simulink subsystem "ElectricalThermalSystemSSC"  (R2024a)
settings: Solver=VariableStepAuto  StartTime=0.0  StopTime=10.0  RelTol=1e-3
undefined symbols (not defined in the file): coolant_pipe_D, coolant_valve_D_ratio_max, coolant_valve_D_ratio_min, coolant_valve_displacement, EnvAirTemp, EnvGrvty, PlantThrEstCmpPwr, PlntThrChArea, PlntThrFanMaxSpd, PlntThrFanMechEff, PlntThrFanVolEff, PlntThrHeaterMaxPwr, PlntThrPipeArea, PlntThrPipeDia, PlntThrPmpMaxSpd, PlntThrRadRamEff, PlntThrRefrigAinit, PlntThrTankArea, PlntThrTankVol, PlntThrValDisp, PlntThrValDratioMax, PlntThrValDratioMin, PlntThrValSplMax, ThrmEM1, ThrmEM2, ThrmEM3, ThrmEM4
libraries: fl_lib x148, nesl_utility x61, SimscapeFluids_lib x25, autolibutils x12
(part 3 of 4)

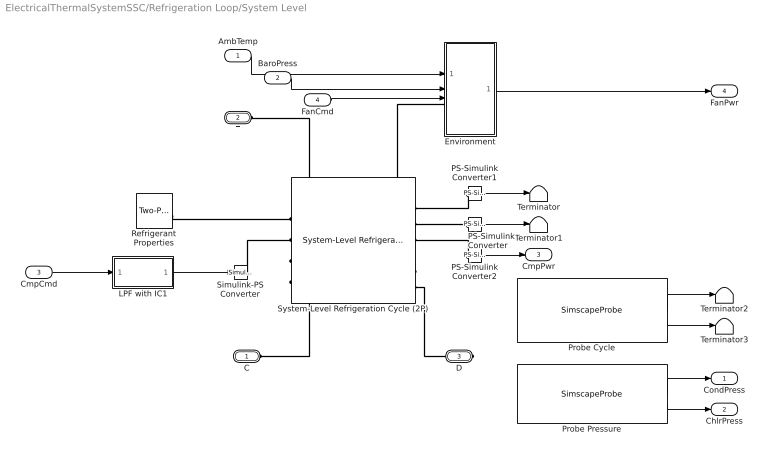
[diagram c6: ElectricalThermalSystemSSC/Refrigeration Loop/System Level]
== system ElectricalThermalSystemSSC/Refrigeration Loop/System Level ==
  AmbTemp : Inport
  BaroPress : Inport  Port=2
  CmpCmd : Inport  Port=3
  FanCmd : Inport  Port=4
  Environment : Subsystem
  LPF with IC1 : Subsystem  mask{wc=0.2, InitCond=0, dataType=off}
      mask prompts: wc "Cutoff frequency, wc [rad/s]"; InitCond "Initial condition, InitCond [same as u]"; dataType "Enforce same input data type"
  PS-Simulink Converter : nesl_utility/PS-Simulink Converter  PhysicalDomain=network_engine_domain  SubClassName=ps_output  LeftPortType=input  RightPortType=output  PseudoPeriodic=off  Frequencies=[]  VectorFormat=inherit  Unit=W  AffineConversion=off
  PS-Simulink Converter1 : nesl_utility/PS-Simulink Converter  PhysicalDomain=network_engine_domain  SubClassName=ps_output  LeftPortType=input  RightPortType=output  PseudoPeriodic=off  Frequencies=[]  VectorFormat=inherit  Unit=W  AffineConversion=off
  PS-Simulink Converter2 : nesl_utility/PS-Simulink Converter  PhysicalDomain=network_engine_domain  SubClassName=ps_output  LeftPortType=input  RightPortType=output  PseudoPeriodic=off  Frequencies=[]  VectorFormat=inherit  Unit=W  AffineConversion=off
  Probe Cycle : SimscapeProbe  BoundBlock=25446  Variables={h_cycle, p_cycle}
  Probe Pressure : SimscapeProbe  BoundBlock=25446  Variables={condenser.refrigerant.p, evaporator.refrigerant.p}
  Refrigerant Properties : SimscapeFluids_lib/Two-Phase Fluid/Utilities/Two-Phase Fluid Predefined Properties (2P)  fluid=fluids.two_phase_fluid.utilities.enum.Fluid.R134a  p_atm=0.101325 MPa  properties_range_check=simscape.enum.assert.action.error  q_rev=0.01 Pa
  Simulink-PS Converter : nesl_utility/Simulink-PS Converter  PhysicalDomain=network_engine_domain  SubClassName=ps_input  LeftPortType=input  RightPortType=output  PseudoPeriodic=off  Frequencies=[]  NoiseDistribution=none  NoiseParameters=[]  Unit=1  AffineConversion=off  FilteringAndDerivatives=provide  SimscapeFilterOrder=1  InputFilterTimeConstant=0.001  UdotUserProvided=0
  System-Level Refrigeration Cycle (2P) : SimscapeFluids_lib/Two-Phase Fluid/Thermodynamic Cycles/System-Level Refrigeration Cycle (2P)  capacity_spec=fluids.two_phase_fluid.thermodynamic_cycles.enum.RefrigerationCycleCapacitySpec.CoolingLoad  Q_cond_nominal=15 kW  Q_evap_nominal=PlntThrCycNomHeatflw kW  mdot_nominal=0.005 kg/s  pressure_spec=fluids.two_phase_fluid.thermodynamic_cycles.enum.RefrigerationCyclePressureSpec.Pressure  p_cond_nominal=PlntThrCycCondRefPin kPa  p_evap_nominal=PlntThrCycChlrRefPin kPa  T_cond_nominal=333.15 K  T_evap_nominal=273.15 K  delta_T_sub_nominal=5 deltaK  delta_T_sup_nominal=10 deltaK  delta_T_sup_static=5 deltaK  performance_spec=fluids.two_phase_fluid.thermodynamic_cycles.enum.RefrigerationCyclePerformanceSpec.COPCooling  COP_nominal=3  comp_eta_s=0.8  comp_eta_v_nominal=0.95  comp_eta_m=0.95  valve_max_fraction=1.5  valve_leak_fraction=1e-6  valve_smoothing_factor=0.01  volume_cond=PlntThrCycCondRefVol m^3  volume_evap=PlntThrCycChlrRefVol m^3  receiver_volume=2 l  receiver_L_init=1 - PlntThrRefrigAinit  nominal_init=true  p_cond_init=refrigerant_p_init MPa  p_evap_init=refrigerant_p_init MPa  h_cond_init=[450, 250] kJ/kg  h_evap_init=[250, 400] kJ/kg  receiver_saturated_init=true  receiver_h_liq_init=500 kJ/kg  receiver_h_vap_init=3500 kJ/kg  cond_domain=fluids.two_phase_fluid.thermodynamic_cycles.enum.RefrigerationCycleFluidDomain.MoistAir  cond_mdot_nominal=PlntThrCycCondAirFlw kg/s  cond_delta_p_nominal=PlntThrCondNomAirDP Pa  cond_pressure_spec=fluids.two_phase_fluid.thermodynamic_cycles.enum.RefrigerationCyclePressureSpec.Pressure  cond_p_in_nominal=PlntThrCondNomPin Pa  cond_T_sat_nominal=400 K  cond_inlet_spec=fluids.two_phase_fluid.thermodynamic_cycles.enum.RefrigerationCycleInletSpec.Enthalpy  cond_T_in_nominal=PlntThrCondNomTin K  cond_h_in_nominal=500 kJ/kg  cond_x_in_nominal=1  cond_inlet_moisture_spec=foundation.enum.moisture_spec.relative_humidity  cond_RH_in_nominal=PlntThrCondNomRelH  cond_x_w_in_nominal=0.01  cond_y_w_in_nominal=0.01  cond_HR_in_nominal=0.01  cond_Tw_in_nominal=287 K  cond_inlet_trace_gas_spec=foundation.enum.trace_gas_spec.mole_fraction  cond_x_g_in_nominal=cabin_CO2_init  cond_y_g_in_nominal=PlntThrCabCO2Init  cond_volume=PlntThrCycCondNomVol m^3  area_Ac=PlntThrCabDucArea m^2  area_Bc=PlntThrCabDucArea m^2  cond_wall_thermal_mass=true  cond_mass_wall=1 kg  cond_cp_wall=890 J/(K*kg)  cond_nominal_init=false  cond_p_init=EnvAbsPrs Pa  cond_energy_spec=foundation.enum.energy_spec.enthalpy  cond_T_init=EnvAirTemp K  cond_x_init=0.5  cond_alpha_init=0.5  cond_h_init=1500 kJ/kg  cond_u_init=1500 kJ/kg  cond_moisture_spec=foundation.enum.moisture_spec.relative_humidity  cond_RH_init=PlntThrCabRelHInit  cond_x_w_init=0.01  cond_y_w_init=0.01  cond_HR_init=0.01  cond_Tw_init=287 K  cond_trace_gas_spec=foundation.enum.trace_gas_spec.mole_fraction  cond_x_g_init=0.001  cond_y_g_init=PlntThrCabCO2Init  cond_T_wall_init=EnvAirTemp K  cond_RH_ws=1  evap_domain=fluids.two_phase_fluid.thermodynamic_cycles.enum.RefrigerationCycleFluidDomain.ThermalLiquid  evap_mdot_nominal=PlntThrCycChlrH2OFlw kg/s  evap_delta_p_nominal=PlntThrCycChlrH2ODP Pa  evap_pressure_spec=fluids.two_phase_fluid.thermodynamic_cycles.enum.RefrigerationCyclePressureSpec.Pressure  evap_p_in_nominal=PlntThrCycChlrH2OPin Pa  evap_T_sat_nominal=400 K  evap_inlet_spec=fluids.two_phase_fluid.thermodynamic_cycles.enum.RefrigerationCycleInletSpec.Enthalpy  evap_T_in_nominal=PlntThrCycChlrH2OTin K  evap_h_in_nominal=500 kJ/kg  evap_x_in_nominal=1  evap_inlet_moisture_spec=foundation.enum.moisture_spec.relative_humidity  evap_RH_in_nominal=0.1  evap_x_w_in_nominal=0.01  evap_y_w_in_nominal=0.01  evap_HR_in_nominal=0.01  evap_Tw_in_nominal=287 K  evap_inlet_trace_gas_spec=foundation.enum.trace_gas_spec.mass_fraction  evap_x_g_in_nominal=0.001  evap_y_g_in_nominal=0.001  evap_volume=PlntThrCycChlrH2OVol m^3  area_Ae=PlntThrPipeArea m^2  area_Be=PlntThrPipeArea m^2  evap_wall_thermal_mass=true  evap_mass_wall=1 kg  evap_cp_wall=890 J/(K*kg)  evap_nominal_init=false  evap_p_init=EnvAbsPrs Pa  evap_energy_spec=foundation.enum.energy_spec.enthalpy  evap_T_init=EnvAirTemp K  evap_x_init=0.5  evap_alpha_init=0.5  evap_h_init=1500 kJ/kg  evap_u_init=1500 kJ/kg  evap_moisture_spec=foundation.enum.moisture_spec.relative_humidity  evap_RH_init=0.5  evap_x_w_init=0.01  evap_y_w_init=0.01  evap_HR_init=0.01  evap_Tw_init=287 K  evap_trace_gas_spec=foundation.enum.trace_gas_spec.mass_fraction  evap_x_g_init=0.001  evap_y_g_init=0.001  evap_T_wall_init=EnvAirTemp K  evap_RH_ws=1  cond_coeff_modify=false  cond_a_liq_refrig=0.023  cond_a_mix_refrig=0.005  cond_a_vap_refrig=0.023  cond_b_refrig=0.8  cond_c_refrig=0.33  cond_a_liq_extfld=0.023  cond_a_mix_extfld=0.005  cond_a_vap_extfld=0.023  cond_a_extfld=0.023  cond_b_extfld=0.8  cond_c_extfld=0.33  evap_coeff_modify=false  evap_a_liq_refrig=0.023  evap_a_mix_refrig=0.005  evap_a_vap_refrig=0.023  evap_b_refrig=0.8  evap_c_refrig=0.33  evap_a_liq_extfld=0.023  evap_a_mix_extfld=0.005  evap_a_vap_extfld=0.023  evap_a_extfld=0.023  evap_b_extfld=0.8  evap_c_extfld=0.33
  Terminator{,1..3} (4 alike) : Terminator
  C : PMIOPort  Side=Left
  T : PMIOPort  Port=2  Side=Left
  D : PMIOPort  Port=3  Side=Right
  CondPress : Outport
  ChlrPress : Outport  Port=2
  CmpPwr : Outport  Port=3
  FanPwr : Outport  Port=4
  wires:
  PS-Simulink Converter2/1 -> CmpPwr/1
  Environment/1(FanPwr) -> FanPwr/1
  FanCmd/1 -> Environment/3(FanCmd)
  AmbTemp/1 -> Environment/1(AmbTemp)
  BaroPress/1 -> Environment/2(BaroPress)
  LPF with IC1/1(y) -> Simulink-PS Converter/1
  Probe Pressure/2 -> ChlrPress/1
  Probe Pressure/1 -> CondPress/1
  Probe Cycle/1 -> Terminator2/1
  Probe Cycle/2 -> Terminator3/1
  CmpCmd/1 -> LPF with IC1/1(u)
  PS-Simulink Converter1/1 -> Terminator/1
  PS-Simulink Converter/1 -> Terminator1/1
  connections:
  PS-Simulink Converter2/LConn1 -- System-Level Refrigeration Cycle (2P)/RConn3
  PS-Simulink Converter1/LConn1 -- System-Level Refrigeration Cycle (2P)/RConn1
  PS-Simulink Converter/LConn1 -- System-Level Refrigeration Cycle (2P)/RConn2
  Simulink-PS Converter/RConn1 -- System-Level Refrigeration Cycle (2P)/LConn2
  C/RConn1 -- System-Level Refrigeration Cycle (2P)/RConn5
  D/RConn1 -- System-Level Refrigeration Cycle (2P)/RConn6
  Environment/LConn1 -- System-Level Refrigeration Cycle (2P)/LConn4
  Refrigerant Properties/RConn1 -- System-Level Refrigeration Cycle (2P)/LConn1
  T/RConn1 -- System-Level Refrigeration Cycle (2P)/LConn3

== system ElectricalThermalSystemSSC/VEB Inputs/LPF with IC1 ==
  u : Inport
  Cont LPF IC : autolibutils/Cont LPF IC  wc=wc  aMode=1  dataType=off
  Initial Condition : Constant  Value=InitCond  SampleTime=-1
  y : Outport
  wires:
  Initial Condition/1 -> Cont LPF IC/2
  u/1 -> Cont LPF IC/1
  Cont LPF IC/1 -> y/1

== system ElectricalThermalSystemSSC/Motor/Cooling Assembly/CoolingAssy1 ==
  CoolEM1 : fl_lib/Thermal/Thermal Elements/Thermal Mass  mass_type=foundation.enum.constant_variable.constant  mass=1 kg  sp_heat=PlntEMCp J/kg/K  mass_min=1e-6 kg  num_ports=foundation.enum.numPorts2.two  m_specify=off  m_priority=High  m=1 kg  m_nominal_specify=off  m_nominal_value=1  m_nominal_unit=kg  T_specify=on  T_priority=High  T=EnvAirTemp K  T_nominal_specify=off  T_nominal_value=1  T_nominal_unit=K  Q_specify=off  Q_priority=None  Q=0 W  Q_nominal_specify=off  Q_nominal_value=1  Q_nominal_unit=W
  Coolant Jacket : SimscapeFluids_lib/Thermal Liquid/Pipes & Fittings/Pipe (TL)  dynamic_compressibility=simscape.enum.onoff.on  inertia=simscape.enum.onoff.off  num_segments=1  pipe_length=PlntThrEMJacLen m  cross_section_geometry=fluids.thermal_liquid.pipes_fittings.enum.CrossSectionGeometry.Custom  pipe_diameter=0.1 m  pipe_inner_diameter=0.05 m  pipe_outer_diameter=0.1 m  pipe_width=0.1 m  pipe_height=0.1 m  pipe_major_axis=0.1 m  pipe_minor_axis=0.05 m  pipe_side=0.1 m  pipe_angle=30 deg  area=PlntThrChArea m^2  Dh=PlntThrChDia m  elevation_spec=foundation.enum.constant_variable.constant  elevation_gain=0 m  gravity_spec=foundation.enum.constant_variable.constant  g=EnvGrvty m/s^2  pressure_loss_spec=fluids.thermal_liquid.pipes_fittings.enum.PressureLossSpec.Haaland  local_pressure_loss_spec=fluids.thermal_liquid.pipes_fittings.enum.LocalLossSpec.AggregateLength  length_add=PlntThrEqLength m  loss_coefficient=0.1  roughness_spec=fluids.thermal_liquid.pipes_fittings.enum.RoughnessSpec.Custom  roughness=1.5e-5 m  Re_friction_TLU=[ 400 1000 1.5e+3 3e+3 4e+3 6e+3 1e+4 2e+4 4e+4 6e+4 1e+5 1e+8 ]  friction_factor_TLU=[ 0.264 0.112 0.07099999999999999 0.0417 0.0387 0.0268 0.025 0.0232 0.0226 0.022 0.0214 0.0214 ]  Re_lam=100  Re_tur=500  shape_factor=64  mdot_nominal=[ 0.1 1 ] kg/s  p_diff_nominal=[ 0.001 0.01 ] MPa  mdot_threshold=1e-6 kg/s  wall_spec=fluids.thermal_liquid.pipes_fittings.enum.wall_spec.rigid  vol_expansion_spec=fluids.thermal_liquid.pipes_fittings.enum.VolumeExpansionSpec.Diameter  area_pressure_gain=1e-6 m^2/MPa  static_pressure_TLU=[.1, 1] MPa  area_pressure_gain_TLU=[1e-05, 1.1e-05] m^2  material_behavior_spec=fluids.thermal_liquid.pipes_fittings.enum.PipeMaterialBehavior.Linear  diameter_pressure_gain=1.2e-6 m/MPa  wall_thickness=0.05 m  elastic_modulus=69 GPa  stress_TLU=[276, 310] MPa  strain_TLU=[.004, .02]  stress_assert_action=simscape.enum.assert.action.none  stress_max=400 MPa  poisson_ratio=0.33  wall_time_constant=0.01 s  thermal_expansion=false  alpha_L_wall=24 um/(deltaK*m)  thermal_expansion_Tref=293.15 K  heat_transfer_spec=fluids.thermal_liquid.pipes_fittings.enum.HeatTransferSpec.DittusBoelter  mdot_nominal_heat=[ 0.1 1 ] kg/s  T_in_nominal=[ 293.15 293.15 ] K  T_out_nominal=[ 300 300 ] K  p_in_nominal_heat=[ 0.101325 0.101325 ] MPa  T_wall_nominal=[ 303.15 303.15 ] K  a_coeff=0.3  b_Re_power=0.8  c_Pr_power=0.33  Nu_lam=3.66  Re_Colburn_TLU=[ 100 150 1000 ]  Colburn_factor_TLU=[ 0.019 0.013 0.002 ]  Re_Nu_TLU=[ 100 150 1000 ]  Pr_Nu_TLU=[ 1 10 ]  Nu_TLU=[ 3.72 4.21; 3.75 4.44; 4.21 7.15 ]  p0_vec=EnvAbsPrs Pa  T0_vec=EnvAirTemp K  mdot0=0.1 kg/s
  PS-Simulink Converter : nesl_utility/PS-Simulink Converter  PhysicalDomain=network_engine_domain  SubClassName=ps_output  LeftPortType=input  RightPortType=output  PseudoPeriodic=off  Frequencies=[]  VectorFormat=1-D array  Unit=K  AffineConversion=on
  Temperature Sensor : fl_lib/Thermal/Thermal Sensors/Temperature Sensor  temperature_measure=foundation.enum.MeasurementReference.difference
  Thermal Reference1 : fl_lib/Thermal/Thermal Elements/Thermal Reference
  H1 : PMIOPort  Side=Right
  A : PMIOPort  Port=2  Side=Left
  B : PMIOPort  Port=3  Side=Right
  EMTemp : Outport
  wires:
  PS-Simulink Converter/1 -> EMTemp/1
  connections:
  Thermal Reference1/LConn1 -- Temperature Sensor/RConn1
  Temperature Sensor/RConn2 -- PS-Simulink Converter/LConn1
  Coolant Jacket/RConn1 -- B/RConn1
  A/RConn1 -- Coolant Jacket/LConn1
  CoolEM1/RConn1 -- Temperature Sensor/LConn1 -- Coolant Jacket/LConn2
  CoolEM1/LConn1 -- H1/RConn1

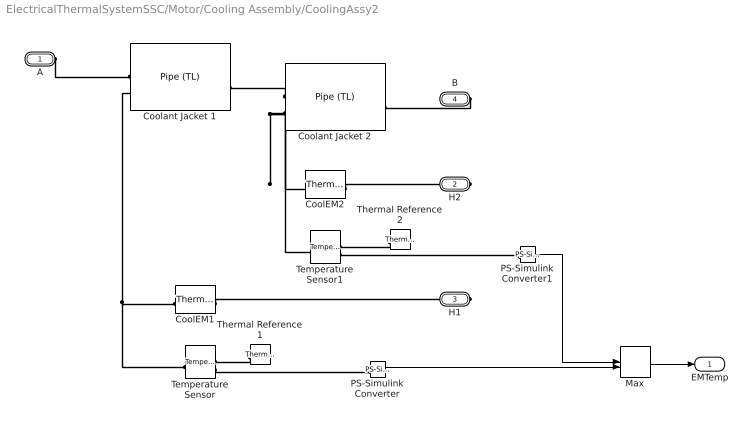
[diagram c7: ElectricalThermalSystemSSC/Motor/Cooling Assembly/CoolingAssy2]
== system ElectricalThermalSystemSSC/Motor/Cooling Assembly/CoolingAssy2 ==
  CoolEM1 : fl_lib/Thermal/Thermal Elements/Thermal Mass  mass_type=foundation.enum.constant_variable.constant  mass=1 kg  sp_heat=PlntEMCp J/kg/K  mass_min=1e-6 kg  num_ports=foundation.enum.numPorts2.two  m_specify=off  m_priority=High  m=1 kg  m_nominal_specify=off  m_nominal_value=1  m_nominal_unit=kg  T_specify=on  T_priority=High  T=EnvAirTemp K  T_nominal_specify=off  T_nominal_value=1  T_nominal_unit=K  Q_specify=off  Q_priority=None  Q=0 W  Q_nominal_specify=off  Q_nominal_value=1  Q_nominal_unit=W
  CoolEM2 : fl_lib/Thermal/Thermal Elements/Thermal Mass  mass_type=foundation.enum.constant_variable.constant  mass=1 kg  sp_heat=PlntEMCp J/kg/K  mass_min=1e-6 kg  num_ports=foundation.enum.numPorts2.two  m_specify=off  m_priority=High  m=1 kg  m_nominal_specify=off  m_nominal_value=1  m_nominal_unit=kg  T_specify=on  T_priority=High  T=EnvAirTemp K  T_nominal_specify=off  T_nominal_value=1  T_nominal_unit=K  Q_specify=off  Q_priority=None  Q=0 W  Q_nominal_specify=off  Q_nominal_value=1  Q_nominal_unit=W
  Coolant Jacket 1 : SimscapeFluids_lib/Thermal Liquid/Pipes & Fittings/Pipe (TL)  dynamic_compressibility=simscape.enum.onoff.on  inertia=simscape.enum.onoff.off  num_segments=1  pipe_length=PlntThrEMJacLen m  cross_section_geometry=fluids.thermal_liquid.pipes_fittings.enum.CrossSectionGeometry.Custom  pipe_diameter=0.1 m  pipe_inner_diameter=0.05 m  pipe_outer_diameter=0.1 m  pipe_width=0.1 m  pipe_height=0.1 m  pipe_major_axis=0.1 m  pipe_minor_axis=0.05 m  pipe_side=0.1 m  pipe_angle=30 deg  area=PlntThrChArea m^2  Dh=PlntThrChDia m  elevation_spec=foundation.enum.constant_variable.constant  elevation_gain=0 m  gravity_spec=foundation.enum.constant_variable.constant  g=EnvGrvty m/s^2  pressure_loss_spec=fluids.thermal_liquid.pipes_fittings.enum.PressureLossSpec.Haaland  local_pressure_loss_spec=fluids.thermal_liquid.pipes_fittings.enum.LocalLossSpec.AggregateLength  length_add=PlntThrEqLength m  loss_coefficient=0.1  roughness_spec=fluids.thermal_liquid.pipes_fittings.enum.RoughnessSpec.Custom  roughness=1.5e-5 m  Re_friction_TLU=[ 400 1000 1.5e+3 3e+3 4e+3 6e+3 1e+4 2e+4 4e+4 6e+4 1e+5 1e+8 ]  friction_factor_TLU=[ 0.264 0.112 0.07099999999999999 0.0417 0.0387 0.0268 0.025 0.0232 0.0226 0.022 0.0214 0.0214 ]  Re_lam=100  Re_tur=500  shape_factor=64  mdot_nominal=[ 0.1 1 ] kg/s  p_diff_nominal=[ 0.001 0.01 ] MPa  mdot_threshold=1e-6 kg/s  wall_spec=fluids.thermal_liquid.pipes_fittings.enum.wall_spec.rigid  vol_expansion_spec=fluids.thermal_liquid.pipes_fittings.enum.VolumeExpansionSpec.Diameter  area_pressure_gain=1e-6 m^2/MPa  static_pressure_TLU=[.1, 1] MPa  area_pressure_gain_TLU=[1e-05, 1.1e-05] m^2  material_behavior_spec=fluids.thermal_liquid.pipes_fittings.enum.PipeMaterialBehavior.Linear  diameter_pressure_gain=1.2e-6 m/MPa  wall_thickness=0.05 m  elastic_modulus=69 GPa  stress_TLU=[276, 310] MPa  strain_TLU=[.004, .02]  stress_assert_action=simscape.enum.assert.action.none  stress_max=400 MPa  poisson_ratio=0.33  wall_time_constant=0.01 s  thermal_expansion=false  alpha_L_wall=24 um/(deltaK*m)  thermal_expansion_Tref=293.15 K  heat_transfer_spec=fluids.thermal_liquid.pipes_fittings.enum.HeatTransferSpec.DittusBoelter  mdot_nominal_heat=[ 0.1 1 ] kg/s  T_in_nominal=[ 293.15 293.15 ] K  T_out_nominal=[ 300 300 ] K  p_in_nominal_heat=[ 0.101325 0.101325 ] MPa  T_wall_nominal=[ 303.15 303.15 ] K  a_coeff=0.3  b_Re_power=0.8  c_Pr_power=0.33  Nu_lam=3.66  Re_Colburn_TLU=[ 100 150 1000 ]  Colburn_factor_TLU=[ 0.019 0.013 0.002 ]  Re_Nu_TLU=[ 100 150 1000 ]  Pr_Nu_TLU=[ 1 10 ]  Nu_TLU=[ 3.72 4.21; 3.75 4.44; 4.21 7.15 ]  p0_vec=EnvAbsPrs Pa  T0_vec=EnvAirTemp K  mdot0=0.1 kg/s
  Coolant Jacket 2 : SimscapeFluids_lib/Thermal Liquid/Pipes & Fittings/Pipe (TL)  dynamic_compressibility=simscape.enum.onoff.on  inertia=simscape.enum.onoff.off  num_segments=1  pipe_length=PlntThrEMJacLen m  cross_section_geometry=fluids.thermal_liquid.pipes_fittings.enum.CrossSectionGeometry.Custom  pipe_diameter=0.1 m  pipe_inner_diameter=0.05 m  pipe_outer_diameter=0.1 m  pipe_width=0.1 m  pipe_height=0.1 m  pipe_major_axis=0.1 m  pipe_minor_axis=0.05 m  pipe_side=0.1 m  pipe_angle=30 deg  area=PlntThrChArea m^2  Dh=PlntThrChDia m  elevation_spec=foundation.enum.constant_variable.constant  elevation_gain=0 m  gravity_spec=foundation.enum.constant_variable.constant  g=EnvGrvty m/s^2  pressure_loss_spec=fluids.thermal_liquid.pipes_fittings.enum.PressureLossSpec.Haaland  local_pressure_loss_spec=fluids.thermal_liquid.pipes_fittings.enum.LocalLossSpec.AggregateLength  length_add=PlntThrEqLength m  loss_coefficient=0.1  roughness_spec=fluids.thermal_liquid.pipes_fittings.enum.RoughnessSpec.Custom  roughness=1.5e-5 m  Re_friction_TLU=[ 400 1000 1.5e+3 3e+3 4e+3 6e+3 1e+4 2e+4 4e+4 6e+4 1e+5 1e+8 ]  friction_factor_TLU=[ 0.264 0.112 0.07099999999999999 0.0417 0.0387 0.0268 0.025 0.0232 0.0226 0.022 0.0214 0.0214 ]  Re_lam=100  Re_tur=500  shape_factor=64  mdot_nominal=[ 0.1 1 ] kg/s  p_diff_nominal=[ 0.001 0.01 ] MPa  mdot_threshold=1e-6 kg/s  wall_spec=fluids.thermal_liquid.pipes_fittings.enum.wall_spec.rigid  vol_expansion_spec=fluids.thermal_liquid.pipes_fittings.enum.VolumeExpansionSpec.Diameter  area_pressure_gain=1e-6 m^2/MPa  static_pressure_TLU=[.1, 1] MPa  area_pressure_gain_TLU=[1e-05, 1.1e-05] m^2  material_behavior_spec=fluids.thermal_liquid.pipes_fittings.enum.PipeMaterialBehavior.Linear  diameter_pressure_gain=1.2e-6 m/MPa  wall_thickness=0.05 m  elastic_modulus=69 GPa  stress_TLU=[276, 310] MPa  strain_TLU=[.004, .02]  stress_assert_action=simscape.enum.assert.action.none  stress_max=400 MPa  poisson_ratio=0.33  wall_time_constant=0.01 s  thermal_expansion=false  alpha_L_wall=24 um/(deltaK*m)  thermal_expansion_Tref=293.15 K  heat_transfer_spec=fluids.thermal_liquid.pipes_fittings.enum.HeatTransferSpec.DittusBoelter  mdot_nominal_heat=[ 0.1 1 ] kg/s  T_in_nominal=[ 293.15 293.15 ] K  T_out_nominal=[ 300 300 ] K  p_in_nominal_heat=[ 0.101325 0.101325 ] MPa  T_wall_nominal=[ 303.15 303.15 ] K  a_coeff=0.3  b_Re_power=0.8  c_Pr_power=0.33  Nu_lam=3.66  Re_Colburn_TLU=[ 100 150 1000 ]  Colburn_factor_TLU=[ 0.019 0.013 0.002 ]  Re_Nu_TLU=[ 100 150 1000 ]  Pr_Nu_TLU=[ 1 10 ]  Nu_TLU=[ 3.72 4.21; 3.75 4.44; 4.21 7.15 ]  p0_vec=EnvAbsPrs Pa  T0_vec=EnvAirTemp K  mdot0=0.1 kg/s
  Max : MinMax  Function=max  Inputs=2
  PS-Simulink Converter : nesl_utility/PS-Simulink Converter  PhysicalDomain=network_engine_domain  SubClassName=ps_output  LeftPortType=input  RightPortType=output  PseudoPeriodic=off  Frequencies=[]  VectorFormat=1-D array  Unit=K  AffineConversion=on
  PS-Simulink Converter1 : nesl_utility/PS-Simulink Converter  PhysicalDomain=network_engine_domain  SubClassName=ps_output  LeftPortType=input  RightPortType=output  PseudoPeriodic=off  Frequencies=[]  VectorFormat=1-D array  Unit=K  AffineConversion=on
  Temperature Sensor : fl_lib/Thermal/Thermal Sensors/Temperature Sensor  temperature_measure=foundation.enum.MeasurementReference.difference
  Temperature Sensor1 : fl_lib/Thermal/Thermal Sensors/Temperature Sensor  temperature_measure=foundation.enum.MeasurementReference.difference
  Thermal Reference1 : fl_lib/Thermal/Thermal Elements/Thermal Reference
  Thermal Reference2 : fl_lib/Thermal/Thermal Elements/Thermal Reference
  A : PMIOPort  Side=Left
  H2 : PMIOPort  Port=2  Side=Right
  H1 : PMIOPort  Port=3  Side=Right
  B : PMIOPort  Port=4  Side=Right
  EMTemp : Outport
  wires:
  PS-Simulink Converter/1 -> Max/2
  PS-Simulink Converter1/1 -> Max/1
  Max/1 -> EMTemp/1
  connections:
  PS-Simulink Converter1/LConn1 -- Temperature Sensor1/RConn2
  Thermal Reference2/LConn1 -- Temperature Sensor1/RConn1
  Coolant Jacket 2/LConn2 -- Temperature Sensor1/LConn1 -- CoolEM2/RConn1
  CoolEM2/LConn1 -- H2/RConn1
  B/RConn1 -- Coolant Jacket 2/RConn1
  Coolant Jacket 2/LConn1 -- Coolant Jacket 1/RConn1
  Thermal Reference1/LConn1 -- Temperature Sensor/RConn1
  Temperature Sensor/RConn2 -- PS-Simulink Converter/LConn1
  A/RConn1 -- Coolant Jacket 1/LConn1
  Temperature Sensor/LConn1 -- Coolant Jacket 1/LConn2 -- CoolEM1/RConn1
  CoolEM1/LConn1 -- H1/RConn1

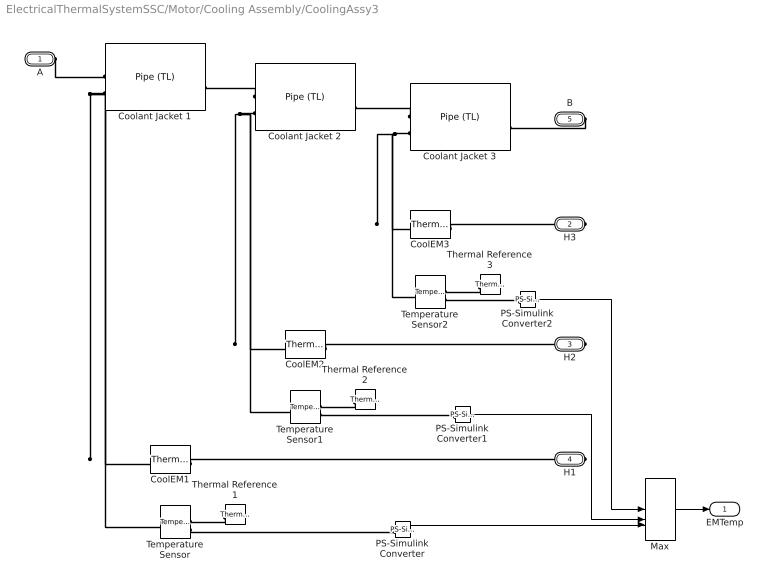
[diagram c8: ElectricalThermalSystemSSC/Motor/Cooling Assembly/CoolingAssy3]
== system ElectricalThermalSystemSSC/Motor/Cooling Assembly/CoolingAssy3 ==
  CoolEM1 : fl_lib/Thermal/Thermal Elements/Thermal Mass  mass_type=foundation.enum.constant_variable.constant  mass=1 kg  sp_heat=PlntEMCp J/kg/K  mass_min=1e-6 kg  num_ports=foundation.enum.numPorts2.two  m_specify=off  m_priority=High  m=1 kg  m_nominal_specify=off  m_nominal_value=1  m_nominal_unit=kg  T_specify=on  T_priority=High  T=EnvAirTemp K  T_nominal_specify=off  T_nominal_value=1  T_nominal_unit=K  Q_specify=off  Q_priority=None  Q=0 W  Q_nominal_specify=off  Q_nominal_value=1  Q_nominal_unit=W
  CoolEM2 : fl_lib/Thermal/Thermal Elements/Thermal Mass  mass_type=foundation.enum.constant_variable.constant  mass=1 kg  sp_heat=PlntEMCp J/kg/K  mass_min=1e-6 kg  num_ports=foundation.enum.numPorts2.two  m_specify=off  m_priority=High  m=1 kg  m_nominal_specify=off  m_nominal_value=1  m_nominal_unit=kg  T_specify=on  T_priority=High  T=EnvAirTemp K  T_nominal_specify=off  T_nominal_value=1  T_nominal_unit=K  Q_specify=off  Q_priority=None  Q=0 W  Q_nominal_specify=off  Q_nominal_value=1  Q_nominal_unit=W
  CoolEM3 : fl_lib/Thermal/Thermal Elements/Thermal Mass  mass_type=foundation.enum.constant_variable.constant  mass=1 kg  sp_heat=PlntEMCp J/kg/K  mass_min=1e-6 kg  num_ports=foundation.enum.numPorts2.two  m_specify=off  m_priority=High  m=1 kg  m_nominal_specify=off  m_nominal_value=1  m_nominal_unit=kg  T_specify=on  T_priority=High  T=EnvAirTemp K  T_nominal_specify=off  T_nominal_value=1  T_nominal_unit=K  Q_specify=off  Q_priority=None  Q=0 W  Q_nominal_specify=off  Q_nominal_value=1  Q_nominal_unit=W
  Coolant Jacket 1 : SimscapeFluids_lib/Thermal Liquid/Pipes & Fittings/Pipe (TL)  dynamic_compressibility=simscape.enum.onoff.on  inertia=simscape.enum.onoff.off  num_segments=1  pipe_length=PlntThrEMJacLen m  cross_section_geometry=fluids.thermal_liquid.pipes_fittings.enum.CrossSectionGeometry.Custom  pipe_diameter=0.1 m  pipe_inner_diameter=0.05 m  pipe_outer_diameter=0.1 m  pipe_width=0.1 m  pipe_height=0.1 m  pipe_major_axis=0.1 m  pipe_minor_axis=0.05 m  pipe_side=0.1 m  pipe_angle=30 deg  area=PlntThrChArea m^2  Dh=PlntThrChDia m  elevation_spec=foundation.enum.constant_variable.constant  elevation_gain=0 m  gravity_spec=foundation.enum.constant_variable.constant  g=EnvGrvty m/s^2  pressure_loss_spec=fluids.thermal_liquid.pipes_fittings.enum.PressureLossSpec.Haaland  local_pressure_loss_spec=fluids.thermal_liquid.pipes_fittings.enum.LocalLossSpec.AggregateLength  length_add=PlntThrEqLength m  loss_coefficient=0.1  roughness_spec=fluids.thermal_liquid.pipes_fittings.enum.RoughnessSpec.Custom  roughness=1.5e-5 m  Re_friction_TLU=[ 400 1000 1.5e+3 3e+3 4e+3 6e+3 1e+4 2e+4 4e+4 6e+4 1e+5 1e+8 ]  friction_factor_TLU=[ 0.264 0.112 0.07099999999999999 0.0417 0.0387 0.0268 0.025 0.0232 0.0226 0.022 0.0214 0.0214 ]  Re_lam=100  Re_tur=500  shape_factor=64  mdot_nominal=[ 0.1 1 ] kg/s  p_diff_nominal=[ 0.001 0.01 ] MPa  mdot_threshold=1e-6 kg/s  wall_spec=fluids.thermal_liquid.pipes_fittings.enum.wall_spec.rigid  vol_expansion_spec=fluids.thermal_liquid.pipes_fittings.enum.VolumeExpansionSpec.Diameter  area_pressure_gain=1e-6 m^2/MPa  static_pressure_TLU=[.1, 1] MPa  area_pressure_gain_TLU=[1e-05, 1.1e-05] m^2  material_behavior_spec=fluids.thermal_liquid.pipes_fittings.enum.PipeMaterialBehavior.Linear  diameter_pressure_gain=1.2e-6 m/MPa  wall_thickness=0.05 m  elastic_modulus=69 GPa  stress_TLU=[276, 310] MPa  strain_TLU=[.004, .02]  stress_assert_action=simscape.enum.assert.action.none  stress_max=400 MPa  poisson_ratio=0.33  wall_time_constant=0.01 s  thermal_expansion=false  alpha_L_wall=24 um/(deltaK*m)  thermal_expansion_Tref=293.15 K  heat_transfer_spec=fluids.thermal_liquid.pipes_fittings.enum.HeatTransferSpec.DittusBoelter  mdot_nominal_heat=[ 0.1 1 ] kg/s  T_in_nominal=[ 293.15 293.15 ] K  T_out_nominal=[ 300 300 ] K  p_in_nominal_heat=[ 0.101325 0.101325 ] MPa  T_wall_nominal=[ 303.15 303.15 ] K  a_coeff=0.3  b_Re_power=0.8  c_Pr_power=0.33  Nu_lam=3.66  Re_Colburn_TLU=[ 100 150 1000 ]  Colburn_factor_TLU=[ 0.019 0.013 0.002 ]  Re_Nu_TLU=[ 100 150 1000 ]  Pr_Nu_TLU=[ 1 10 ]  Nu_TLU=[ 3.72 4.21; 3.75 4.44; 4.21 7.15 ]  p0_vec=EnvAbsPrs Pa  T0_vec=EnvAirTemp K  mdot0=0.1 kg/s
  Coolant Jacket 2 : SimscapeFluids_lib/Thermal Liquid/Pipes & Fittings/Pipe (TL)  dynamic_compressibility=simscape.enum.onoff.on  inertia=simscape.enum.onoff.off  num_segments=1  pipe_length=PlntThrEMJacLen m  cross_section_geometry=fluids.thermal_liquid.pipes_fittings.enum.CrossSectionGeometry.Custom  pipe_diameter=0.1 m  pipe_inner_diameter=0.05 m  pipe_outer_diameter=0.1 m  pipe_width=0.1 m  pipe_height=0.1 m  pipe_major_axis=0.1 m  pipe_minor_axis=0.05 m  pipe_side=0.1 m  pipe_angle=30 deg  area=PlntThrChArea m^2  Dh=PlntThrChDia m  elevation_spec=foundation.enum.constant_variable.constant  elevation_gain=0 m  gravity_spec=foundation.enum.constant_variable.constant  g=EnvGrvty m/s^2  pressure_loss_spec=fluids.thermal_liquid.pipes_fittings.enum.PressureLossSpec.Haaland  local_pressure_loss_spec=fluids.thermal_liquid.pipes_fittings.enum.LocalLossSpec.AggregateLength  length_add=PlntThrEqLength m  loss_coefficient=0.1  roughness_spec=fluids.thermal_liquid.pipes_fittings.enum.RoughnessSpec.Custom  roughness=1.5e-5 m  Re_friction_TLU=[ 400 1000 1.5e+3 3e+3 4e+3 6e+3 1e+4 2e+4 4e+4 6e+4 1e+5 1e+8 ]  friction_factor_TLU=[ 0.264 0.112 0.07099999999999999 0.0417 0.0387 0.0268 0.025 0.0232 0.0226 0.022 0.0214 0.0214 ]  Re_lam=100  Re_tur=500  shape_factor=64  mdot_nominal=[ 0.1 1 ] kg/s  p_diff_nominal=[ 0.001 0.01 ] MPa  mdot_threshold=1e-6 kg/s  wall_spec=fluids.thermal_liquid.pipes_fittings.enum.wall_spec.rigid  vol_expansion_spec=fluids.thermal_liquid.pipes_fittings.enum.VolumeExpansionSpec.Diameter  area_pressure_gain=1e-6 m^2/MPa  static_pressure_TLU=[.1, 1] MPa  area_pressure_gain_TLU=[1e-05, 1.1e-05] m^2  material_behavior_spec=fluids.thermal_liquid.pipes_fittings.enum.PipeMaterialBehavior.Linear  diameter_pressure_gain=1.2e-6 m/MPa  wall_thickness=0.05 m  elastic_modulus=69 GPa  stress_TLU=[276, 310] MPa  strain_TLU=[.004, .02]  stress_assert_action=simscape.enum.assert.action.none  stress_max=400 MPa  poisson_ratio=0.33  wall_time_constant=0.01 s  thermal_expansion=false  alpha_L_wall=24 um/(deltaK*m)  thermal_expansion_Tref=293.15 K  heat_transfer_spec=fluids.thermal_liquid.pipes_fittings.enum.HeatTransferSpec.DittusBoelter  mdot_nominal_heat=[ 0.1 1 ] kg/s  T_in_nominal=[ 293.15 293.15 ] K  T_out_nominal=[ 300 300 ] K  p_in_nominal_heat=[ 0.101325 0.101325 ] MPa  T_wall_nominal=[ 303.15 303.15 ] K  a_coeff=0.3  b_Re_power=0.8  c_Pr_power=0.33  Nu_lam=3.66  Re_Colburn_TLU=[ 100 150 1000 ]  Colburn_factor_TLU=[ 0.019 0.013 0.002 ]  Re_Nu_TLU=[ 100 150 1000 ]  Pr_Nu_TLU=[ 1 10 ]  Nu_TLU=[ 3.72 4.21; 3.75 4.44; 4.21 7.15 ]  p0_vec=EnvAbsPrs Pa  T0_vec=EnvAirTemp K  mdot0=0.1 kg/s
  Coolant Jacket 3 : SimscapeFluids_lib/Thermal Liquid/Pipes & Fittings/Pipe (TL)  dynamic_compressibility=simscape.enum.onoff.on  inertia=simscape.enum.onoff.off  num_segments=1  pipe_length=PlntThrEMJacLen m  cross_section_geometry=fluids.thermal_liquid.pipes_fittings.enum.CrossSectionGeometry.Custom  pipe_diameter=0.1 m  pipe_inner_diameter=0.05 m  pipe_outer_diameter=0.1 m  pipe_width=0.1 m  pipe_height=0.1 m  pipe_major_axis=0.1 m  pipe_minor_axis=0.05 m  pipe_side=0.1 m  pipe_angle=30 deg  area=PlntThrChArea m^2  Dh=PlntThrChDia m  elevation_spec=foundation.enum.constant_variable.constant  elevation_gain=0 m  gravity_spec=foundation.enum.constant_variable.constant  g=EnvGrvty m/s^2  pressure_loss_spec=fluids.thermal_liquid.pipes_fittings.enum.PressureLossSpec.Haaland  local_pressure_loss_spec=fluids.thermal_liquid.pipes_fittings.enum.LocalLossSpec.AggregateLength  length_add=PlntThrEqLength m  loss_coefficient=0.1  roughness_spec=fluids.thermal_liquid.pipes_fittings.enum.RoughnessSpec.Custom  roughness=1.5e-5 m  Re_friction_TLU=[ 400 1000 1.5e+3 3e+3 4e+3 6e+3 1e+4 2e+4 4e+4 6e+4 1e+5 1e+8 ]  friction_factor_TLU=[ 0.264 0.112 0.07099999999999999 0.0417 0.0387 0.0268 0.025 0.0232 0.0226 0.022 0.0214 0.0214 ]  Re_lam=100  Re_tur=500  shape_factor=64  mdot_nominal=[ 0.1 1 ] kg/s  p_diff_nominal=[ 0.001 0.01 ] MPa  mdot_threshold=1e-6 kg/s  wall_spec=fluids.thermal_liquid.pipes_fittings.enum.wall_spec.rigid  vol_expansion_spec=fluids.thermal_liquid.pipes_fittings.enum.VolumeExpansionSpec.Diameter  area_pressure_gain=1e-6 m^2/MPa  static_pressure_TLU=[.1, 1] MPa  area_pressure_gain_TLU=[1e-05, 1.1e-05] m^2  material_behavior_spec=fluids.thermal_liquid.pipes_fittings.enum.PipeMaterialBehavior.Linear  diameter_pressure_gain=1.2e-6 m/MPa  wall_thickness=0.05 m  elastic_modulus=69 GPa  stress_TLU=[276, 310] MPa  strain_TLU=[.004, .02]  stress_assert_action=simscape.enum.assert.action.none  stress_max=400 MPa  poisson_ratio=0.33  wall_time_constant=0.01 s  thermal_expansion=false  alpha_L_wall=24 um/(deltaK*m)  thermal_expansion_Tref=293.15 K  heat_transfer_spec=fluids.thermal_liquid.pipes_fittings.enum.HeatTransferSpec.DittusBoelter  mdot_nominal_heat=[ 0.1 1 ] kg/s  T_in_nominal=[ 293.15 293.15 ] K  T_out_nominal=[ 300 300 ] K  p_in_nominal_heat=[ 0.101325 0.101325 ] MPa  T_wall_nominal=[ 303.15 303.15 ] K  a_coeff=0.3  b_Re_power=0.8  c_Pr_power=0.33  Nu_lam=3.66  Re_Colburn_TLU=[ 100 150 1000 ]  Colburn_factor_TLU=[ 0.019 0.013 0.002 ]  Re_Nu_TLU=[ 100 150 1000 ]  Pr_Nu_TLU=[ 1 10 ]  Nu_TLU=[ 3.72 4.21; 3.75 4.44; 4.21 7.15 ]  p0_vec=EnvAbsPrs Pa  T0_vec=EnvAirTemp K  mdot0=0.1 kg/s
  Max : MinMax  Function=max  Inputs=3
  PS-Simulink Converter : nesl_utility/PS-Simulink Converter  PhysicalDomain=network_engine_domain  SubClassName=ps_output  LeftPortType=input  RightPortType=output  PseudoPeriodic=off  Frequencies=[]  VectorFormat=1-D array  Unit=K  AffineConversion=on
  PS-Simulink Converter1 : nesl_utility/PS-Simulink Converter  PhysicalDomain=network_engine_domain  SubClassName=ps_output  LeftPortType=input  RightPortType=output  PseudoPeriodic=off  Frequencies=[]  VectorFormat=1-D array  Unit=K  AffineConversion=on
  PS-Simulink Converter2 : nesl_utility/PS-Simulink Converter  PhysicalDomain=network_engine_domain  SubClassName=ps_output  LeftPortType=input  RightPortType=output  PseudoPeriodic=off  Frequencies=[]  VectorFormat=1-D array  Unit=K  AffineConversion=on
  Temperature Sensor : fl_lib/Thermal/Thermal Sensors/Temperature Sensor  temperature_measure=foundation.enum.MeasurementReference.difference
  Temperature Sensor1 : fl_lib/Thermal/Thermal Sensors/Temperature Sensor  temperature_measure=foundation.enum.MeasurementReference.difference
  Temperature Sensor2 : fl_lib/Thermal/Thermal Sensors/Temperature Sensor  temperature_measure=foundation.enum.MeasurementReference.difference
  Thermal Reference1 : fl_lib/Thermal/Thermal Elements/Thermal Reference
  Thermal Reference2 : fl_lib/Thermal/Thermal Elements/Thermal Reference
  Thermal Reference3 : fl_lib/Thermal/Thermal Elements/Thermal Reference
  A : PMIOPort  Side=Left
  H3 : PMIOPort  Port=2  Side=Right
  H2 : PMIOPort  Port=3  Side=Right
  H1 : PMIOPort  Port=4  Side=Right
  B : PMIOPort  Port=5  Side=Right
  EMTemp : Outport
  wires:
  PS-Simulink Converter2/1 -> Max/1
  PS-Simulink Converter1/1 -> Max/2
  PS-Simulink Converter/1 -> Max/3
  Max/1 -> EMTemp/1
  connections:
  Coolant Jacket 3/LConn2 -- Temperature Sensor2/LConn1 -- CoolEM3/RConn1
  B/RConn1 -- Coolant Jacket 3/RConn1
  Coolant Jacket 3/LConn1 -- Coolant Jacket 2/RConn1
  Thermal Reference3/LConn1 -- Temperature Sensor2/RConn1
  PS-Simulink Converter2/LConn1 -- Temperature Sensor2/RConn2
  CoolEM3/LConn1 -- H3/RConn1
  PS-Simulink Converter1/LConn1 -- Temperature Sensor1/RConn2
  Thermal Reference2/LConn1 -- Temperature Sensor1/RConn1
  Coolant Jacket 2/LConn2 -- Temperature Sensor1/LConn1 -- CoolEM2/RConn1
  CoolEM2/LConn1 -- H2/RConn1
  Coolant Jacket 2/LConn1 -- Coolant Jacket 1/RConn1
  Thermal Reference1/LConn1 -- Temperature Sensor/RConn1
  Temperature Sensor/RConn2 -- PS-Simulink Converter/LConn1
  A/RConn1 -- Coolant Jacket 1/LConn1
  Coolant Jacket 1/LConn2 -- CoolEM1/RConn1 -- Temperature Sensor/LConn1
  CoolEM1/LConn1 -- H1/RConn1

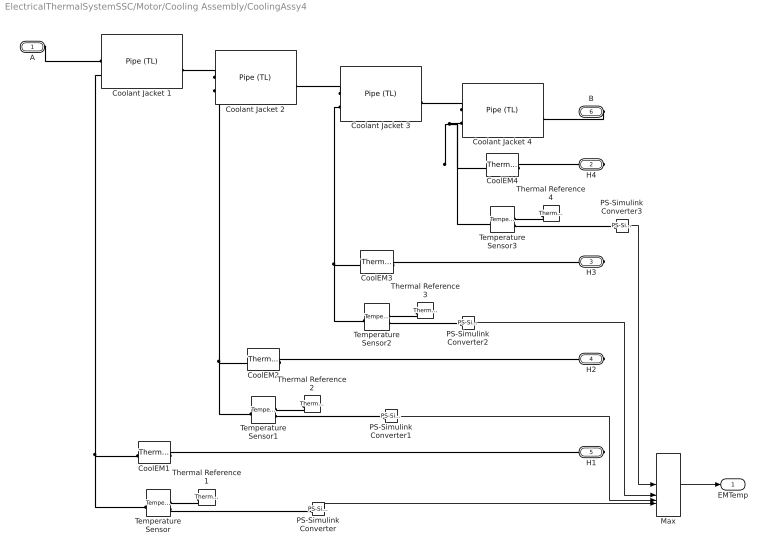
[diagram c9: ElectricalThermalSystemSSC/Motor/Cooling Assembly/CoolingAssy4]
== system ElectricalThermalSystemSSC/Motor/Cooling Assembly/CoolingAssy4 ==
  CoolEM{1..4} (4 alike) : fl_lib/Thermal/Thermal Elements/Thermal Mass  mass_type=foundation.enum.constant_variable.constant  mass=1 kg  sp_heat=PlntEMCp J/kg/K  mass_min=1e-6 kg  num_ports=foundation.enum.numPorts2.two  m_specify=off  m_priority=High  m=1 kg  m_nominal_specify=off  m_nominal_value=1  m_nominal_unit=kg  T_specify=on  T_priority=High  T=EnvAirTemp K  T_nominal_specify=off  T_nominal_value=1  T_nominal_unit=K  Q_specify=off  Q_priority=None  Q=0 W  Q_nominal_specify=off  Q_nominal_value=1  Q_nominal_unit=W
  Coolant Jacket {1..4} (4 alike) : SimscapeFluids_lib/Thermal Liquid/Pipes & Fittings/Pipe (TL)  dynamic_compressibility=simscape.enum.onoff.on  inertia=simscape.enum.onoff.off  num_segments=1  pipe_length=PlntThrEMJacLen m  cross_section_geometry=fluids.thermal_liquid.pipes_fittings.enum.CrossSectionGeometry.Custom  pipe_diameter=0.1 m  pipe_inner_diameter=0.05 m  pipe_outer_diameter=0.1 m  pipe_width=0.1 m  pipe_height=0.1 m  pipe_major_axis=0.1 m  pipe_minor_axis=0.05 m  pipe_side=0.1 m  pipe_angle=30 deg  area=PlntThrChArea m^2  Dh=PlntThrChDia m  elevation_spec=foundation.enum.constant_variable.constant  elevation_gain=0 m  gravity_spec=foundation.enum.constant_variable.constant  g=EnvGrvty m/s^2  pressure_loss_spec=fluids.thermal_liquid.pipes_fittings.enum.PressureLossSpec.Haaland  local_pressure_loss_spec=fluids.thermal_liquid.pipes_fittings.enum.LocalLossSpec.AggregateLength  length_add=PlntThrEqLength m  loss_coefficient=0.1  roughness_spec=fluids.thermal_liquid.pipes_fittings.enum.RoughnessSpec.Custom  roughness=1.5e-5 m  Re_friction_TLU=[ 400 1000 1.5e+3 3e+3 4e+3 6e+3 1e+4 2e+4 4e+4 6e+4 1e+5 1e+8 ]  friction_factor_TLU=[ 0.264 0.112 0.07099999999999999 0.0417 0.0387 0.0268 0.025 0.0232 0.0226 0.022 0.0214 0.0214 ]  Re_lam=100  Re_tur=500  shape_factor=64  mdot_nominal=[ 0.1 1 ] kg/s  p_diff_nominal=[ 0.001 0.01 ] MPa  mdot_threshold=1e-6 kg/s  wall_spec=fluids.thermal_liquid.pipes_fittings.enum.wall_spec.rigid  vol_expansion_spec=fluids.thermal_liquid.pipes_fittings.enum.VolumeExpansionSpec.Diameter  area_pressure_gain=1e-6 m^2/MPa  static_pressure_TLU=[.1, 1] MPa  area_pressure_gain_TLU=[1e-05, 1.1e-05] m^2  material_behavior_spec=fluids.thermal_liquid.pipes_fittings.enum.PipeMaterialBehavior.Linear  diameter_pressure_gain=1.2e-6 m/MPa  wall_thickness=0.05 m  elastic_modulus=69 GPa  stress_TLU=[276, 310] MPa  strain_TLU=[.004, .02]  stress_assert_action=simscape.enum.assert.action.none  stress_max=400 MPa  poisson_ratio=0.33  wall_time_constant=0.01 s  thermal_expansion=false  alpha_L_wall=24 um/(deltaK*m)  thermal_expansion_Tref=293.15 K  heat_transfer_spec=fluids.thermal_liquid.pipes_fittings.enum.HeatTransferSpec.DittusBoelter  mdot_nominal_heat=[ 0.1 1 ] kg/s  T_in_nominal=[ 293.15 293.15 ] K  T_out_nominal=[ 300 300 ] K  p_in_nominal_heat=[ 0.101325 0.101325 ] MPa  T_wall_nominal=[ 303.15 303.15 ] K  a_coeff=0.3  b_Re_power=0.8  c_Pr_power=0.33  Nu_lam=3.66  Re_Colburn_TLU=[ 100 150 1000 ]  Colburn_factor_TLU=[ 0.019 0.013 0.002 ]  Re_Nu_TLU=[ 100 150 1000 ]  Pr_Nu_TLU=[ 1 10 ]  Nu_TLU=[ 3.72 4.21; 3.75 4.44; 4.21 7.15 ]  p0_vec=EnvAbsPrs Pa  T0_vec=EnvAirTemp K  mdot0=0.1 kg/s
  Max : MinMax  Function=max  Inputs=4
  PS-Simulink Converter{,1..3} (4 alike) : nesl_utility/PS-Simulink Converter  PhysicalDomain=network_engine_domain  SubClassName=ps_output  LeftPortType=input  RightPortType=output  PseudoPeriodic=off  Frequencies=[]  VectorFormat=1-D array  Unit=K  AffineConversion=on
  Temperature Sensor{,1..3} (4 alike) : fl_lib/Thermal/Thermal Sensors/Temperature Sensor  temperature_measure=foundation.enum.MeasurementReference.difference
  Thermal Reference{1..4} (4 alike) : fl_lib/Thermal/Thermal Elements/Thermal Reference
  A : PMIOPort  Side=Left
  H4 : PMIOPort  Port=2  Side=Right
  H3 : PMIOPort  Port=3  Side=Right
  H2 : PMIOPort  Port=4  Side=Right
  H1 : PMIOPort  Port=5  Side=Right
  B : PMIOPort  Port=6  Side=Right
  EMTemp : Outport
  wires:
  PS-Simulink Converter3/1 -> Max/1
  PS-Simulink Converter2/1 -> Max/2
  PS-Simulink Converter1/1 -> Max/3
  PS-Simulink Converter/1 -> Max/4
  Max/1 -> EMTemp/1
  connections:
  Coolant Jacket 4/LConn2 -- CoolEM4/RConn1 -- Temperature Sensor3/LConn1
  PS-Simulink Converter3/LConn1 -- Temperature Sensor3/RConn2
  Thermal Reference4/LConn1 -- Temperature Sensor3/RConn1
  CoolEM4/LConn1 -- H4/RConn1
  B/RConn1 -- Coolant Jacket 4/RConn1
  Coolant Jacket 4/LConn1 -- Coolant Jacket 3/RConn1
  Temperature Sensor2/LConn1 -- Coolant Jacket 3/LConn2 -- CoolEM3/RConn1
  Coolant Jacket 3/LConn1 -- Coolant Jacket 2/RConn1
  Thermal Reference3/LConn1 -- Temperature Sensor2/RConn1
  PS-Simulink Converter2/LConn1 -- Temperature Sensor2/RConn2
  CoolEM3/LConn1 -- H3/RConn1
  PS-Simulink Converter1/LConn1 -- Temperature Sensor1/RConn2
  Thermal Reference2/LConn1 -- Temperature Sensor1/RConn1
  Temperature Sensor1/LConn1 -- Coolant Jacket 2/LConn2 -- CoolEM2/RConn1
  CoolEM2/LConn1 -- H2/RConn1
  Coolant Jacket 2/LConn1 -- Coolant Jacket 1/RConn1
  Thermal Reference1/LConn1 -- Temperature Sensor/RConn1
  Temperature Sensor/RConn2 -- PS-Simulink Converter/LConn1
  A/RConn1 -- Coolant Jacket 1/LConn1
  Temperature Sensor/LConn1 -- Coolant Jacket 1/LConn2 -- CoolEM1/RConn1
  CoolEM1/LConn1 -- H1/RConn1

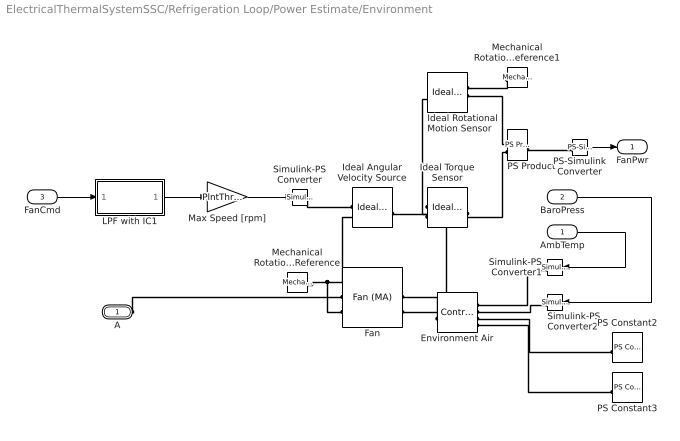
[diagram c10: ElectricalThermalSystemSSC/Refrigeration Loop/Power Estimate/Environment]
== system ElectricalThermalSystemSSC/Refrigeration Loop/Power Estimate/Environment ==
  AmbTemp : Inport
  BaroPress : Inport  Port=2
  FanCmd : Inport  Port=3
  Environment Air : fl_lib/Moist Air/Elements/Controlled Reservoir (MA)  moisture_spec=foundation.enum.moisture_spec.relative_humidity  trace_gas_spec=foundation.enum.trace_gas_spec.mole_fraction  RH_ws=1  area_A=PlntThrRadFanAreaFlw m^2  input_error_spec=foundation.enum.input_range_error.warn
  Fan : SimscapeFluids_lib/Moist Air/Turbomachinery/Fan (MA)  fan_parameterization=fluids.moist_air.turbomachinery.enum.FanParameterization.Nominal  mechanical_power_spec=fluids.moist_air.turbomachinery.enum.FanMechanicalPowerSpec.Efficiency  flow_rate_nominal=0.8 m^3/s  pressure_nominal=PlntThrFanNomP Pa  eta_nominal=PlntThrFanVolEff*PlntThrFanMechEff  power_nominal=1620 W  pressure_max=600 Pa  flow_rate_max=1.5 m^3/s  omega_ref_nominal=1000 rpm  flow_rate_1D_TLU=[.0278, .0556, .0833, .111, .139, .167] m^3/s  pressure_1D_TLU=[6410, 6375, 6018, 5366, 4501, 3609] Pa  eta_1D_TLU=[.257, .394, .453, .47, .459, .415]  power_1D_TLU=[693, 900, 1107, 1267, 1363, 1452] W  omega_ref_1D=3000 rpm  rho_ref_1D=1.2 kg/m^3  omega_threshold_factor=1e-2  omega_dp_TLU=[2400; 3000; 3600] rpm  flow_rate_dp_TLU=[.0278, .0556, .0833, .111, .139, .167] m^3/s  pressure_dp_TLU=[4111, 4010, 3551, 2881, 2167, 1453; 6410, 6375, 6018, 5366, 4501, 3609; 9217, 9285, 9022, 8428, 7552, 6482] Pa  eta_dp_TLU=[.3, .434, .468, .459, .4, .3; .257, .394, .453, .47, .459, .415; .225, .359, .434, .461, .47, .459]  power_dp_TLU=[381, 514, 632, 697, 753, 809; 693, 900, 1107, 1267, 1363, 1452; 1139, 1438, 1732, 2029, 2233, 2358] W  rho_ref_dp=1.2 kg/m^3  omega_q_TLU=[2990; 3450; 3867] rpm  pressure_q_TLU=[31, 62, 93, 124] Pa  flow_rate_q_TLU=[.802, .759, .703, .611; .936, .902, .862, .81; 1.056, 1.027, .994, .956] m^3/s  eta_q_TLU=[.088, .162, .22, .261; .068, .128, .18, .222; .055, .105, .148, .188]  power_q_TLU=[283, 290, 297, 290; 427, 437, 445, 452; 595, 606, 625, 631] W  rho_ref_q=1.2 kg/m^3  diameter_ratio=1  mech_orientation=fluids.moist_air.turbomachinery.enum.FanMechanicalOrientation.Positive  area_A=PlntThrRadFanAreaFlw m^2  area_B=PlntThrRadFanAreaFlw m^2
  Ideal Angular Velocity Source : fl_lib/Mechanical/Mechanical Sources/Ideal Angular Velocity Source
  Ideal Rotational Motion Sensor : fl_lib/Mechanical/Mechanical Sensors/Ideal Rotational Motion Sensor  reference=foundation.enum.MeasurementReference.difference  acceleration_port=false  velocity_port=true  position_port=true  wrap_angle=false  offset=0 rad
  Ideal Torque Sensor : fl_lib/Mechanical/Mechanical Sensors/Ideal Torque Sensor
  LPF with IC1 : Subsystem  mask{wc=0.2, InitCond=0, dataType=off}
      mask prompts: wc "Cutoff frequency, wc [rad/s]"; InitCond "Initial condition, InitCond [same as u]"; dataType "Enforce same input data type"
  Max Speed [rpm] : Gain  Gain=PlntThrFanMaxSpd
  Mechanical Rotational Reference : fl_lib/Mechanical/Rotational Elements/Mechanical Rotational Reference
  Mechanical Rotational Reference1 : fl_lib/Mechanical/Rotational Elements/Mechanical Rotational Reference
  PS Constant2 : fl_lib/Physical Signals/Sources/PS Constant  constant=PlntThrCabRelHInit
  PS Constant3 : fl_lib/Physical Signals/Sources/PS Constant  constant=PlntThrCabCO2Init
  PS Product : fl_lib/Physical Signals/Functions/PS Product
  PS-Simulink Converter : nesl_utility/PS-Simulink Converter  PhysicalDomain=network_engine_domain  SubClassName=ps_output  LeftPortType=input  RightPortType=output  PseudoPeriodic=off  Frequencies=[]  VectorFormat=inherit  Unit=W  AffineConversion=off
  Simulink-PS Converter : nesl_utility/Simulink-PS Converter  PhysicalDomain=network_engine_domain  SubClassName=ps_input  LeftPortType=input  RightPortType=output  PseudoPeriodic=off  Frequencies=[]  NoiseDistribution=none  NoiseParameters=[]  Unit=rpm  AffineConversion=off  FilteringAndDerivatives=provide  SimscapeFilterOrder=1  InputFilterTimeConstant=0.001  UdotUserProvided=0
  Simulink-PS Converter1 : nesl_utility/Simulink-PS Converter  PhysicalDomain=network_engine_domain  SubClassName=ps_input  LeftPortType=input  RightPortType=output  PseudoPeriodic=off  Frequencies=[]  NoiseDistribution=none  NoiseParameters=[]  Unit=K  AffineConversion=on  FilteringAndDerivatives=provide  SimscapeFilterOrder=1  InputFilterTimeConstant=0.001  UdotUserProvided=0
  Simulink-PS Converter2 : nesl_utility/Simulink-PS Converter  PhysicalDomain=network_engine_domain  SubClassName=ps_input  LeftPortType=input  RightPortType=output  PseudoPeriodic=off  Frequencies=[]  NoiseDistribution=none  NoiseParameters=[]  Unit=Pa  AffineConversion=off  FilteringAndDerivatives=provide  SimscapeFilterOrder=1  InputFilterTimeConstant=0.001  UdotUserProvided=0
  A : PMIOPort  Side=Left
  FanPwr : Outport
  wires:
  LPF with IC1/1(y) -> Max Speed [rpm]/1
  FanCmd/1 -> LPF with IC1/1(u)
  Max Speed [rpm]/1 -> Simulink-PS Converter/1
  BaroPress/1 -> Simulink-PS Converter2/1
  PS-Simulink Converter/1 -> FanPwr/1
  AmbTemp/1 -> Simulink-PS Converter1/1
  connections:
  Environment Air/LConn1 -- Fan/RConn1
  Environment Air/RConn3 -- PS Constant2/RConn1
  A/RConn1 -- Fan/LConn1
  Mechanical Rotational Reference1/LConn1 -- Ideal Rotational Motion Sensor/RConn1
  PS Product/LConn2 -- Ideal Torque Sensor/RConn2
  PS Constant3/RConn1 -- Environment Air/RConn4
  Simulink-PS Converter/RConn1 -- Ideal Angular Velocity Source/RConn1
  Simulink-PS Converter1/RConn1 -- Environment Air/RConn1
  Simulink-PS Converter2/RConn1 -- Environment Air/RConn2
  PS-Simulink Converter/LConn1 -- PS Product/RConn1
  Ideal Torque Sensor/RConn1 -- Fan/RConn2
  PS Product/LConn1 -- Ideal Rotational Motion Sensor/RConn2
  Fan/LConn2 -- Ideal Angular Velocity Source/RConn2 -- Mechanical Rotational Reference/LConn1
  Ideal Torque Sensor/LConn1 -- Ideal Rotational Motion Sensor/LConn1 -- Ideal Angular Velocity Source/LConn1

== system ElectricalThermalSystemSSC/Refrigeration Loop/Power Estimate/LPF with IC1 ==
  u : Inport
  Cont LPF IC : autolibutils/Cont LPF IC  wc=wc  aMode=1  dataType=off
  Initial Condition : Constant  Value=InitCond  SampleTime=-1
  y : Outport
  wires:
  Initial Condition/1 -> Cont LPF IC/2
  u/1 -> Cont LPF IC/1
  Cont LPF IC/1 -> y/1

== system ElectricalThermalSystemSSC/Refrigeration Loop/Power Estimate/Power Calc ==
  Input : Inport
  COP : fl_lib/Physical Signals/Lookup Tables/PS Lookup Table (1D)  x=PlntThrEstDTLut deltaK  f=PlntThrEstCOPLut  interp_method=simscape.enum.interpolation.linear  extrap_method=simscape.enum.extrapolation.nearest
  PS Gain : fl_lib/Physical Signals/Functions/PS Gain  gain=-1
  Power Comp : fl_lib/Physical Signals/Functions/PS Gain  gain=PlantThrEstCmpPwr kW
  Power Cond : fl_lib/Physical Signals/Functions/PS Add
  Power Evap : fl_lib/Physical Signals/Functions/PS Product
  Pressure & Temperature Sensor (MA) : fl_lib/Moist Air/Sensors/Pressure & Temperature Sensor (MA)  reference=foundation.enum.MeasurementReference.absolute  pressure=false  pressure_spec=foundation.enum.PressureMeasementSpec.Absolute  temperature=true
  Pressure & Temperature Sensor (TL) : fl_lib/Thermal Liquid/Sensors/Pressure & Temperature Sensor (TL)  reference=foundation.enum.MeasurementReference.absolute  pressure=false  pressure_spec=foundation.enum.PressureMeasementSpec.Absolute  temperature=true
  Simulink-PS Converter : nesl_utility/Simulink-PS Converter  PhysicalDomain=network_engine_domain  SubClassName=ps_input  LeftPortType=input  RightPortType=output  PseudoPeriodic=off  Frequencies=[]  NoiseDistribution=none  NoiseParameters=[]  Unit=1  AffineConversion=off  FilteringAndDerivatives=provide  SimscapeFilterOrder=1  InputFilterTimeConstant=0.001  UdotUserProvided=0
  dT : fl_lib/Physical Signals/Functions/PS Subtract
  Cond : PMIOPort  Side=Left
  MA : PMIOPort  Port=2  Side=Left
  Evap : PMIOPort  Port=3  Side=Right
  TL : PMIOPort  Port=4  Side=Right
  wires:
  Input/1 -> Simulink-PS Converter/1
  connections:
  Power Cond/LConn2 -- PS Gain/LConn1 -- Power Evap/RConn1
  Power Evap/LConn1 -- COP/RConn1
  dT/RConn1 -- COP/LConn1
  Power Evap/LConn2 -- Power Cond/LConn1 -- Power Comp/RConn1
  dT/LConn1 -- Pressure & Temperature Sensor (MA)/RConn1
  Pressure & Temperature Sensor (TL)/RConn1 -- dT/LConn2
  TL/RConn1 -- Pressure & Temperature Sensor (TL)/LConn1
  Simulink-PS Converter/RConn1 -- Power Comp/LConn1
  Pressure & Temperature Sensor (MA)/LConn1 -- MA/RConn1
  Power Cond/RConn1 -- Cond/RConn1
  Evap/RConn1 -- PS Gain/RConn1
